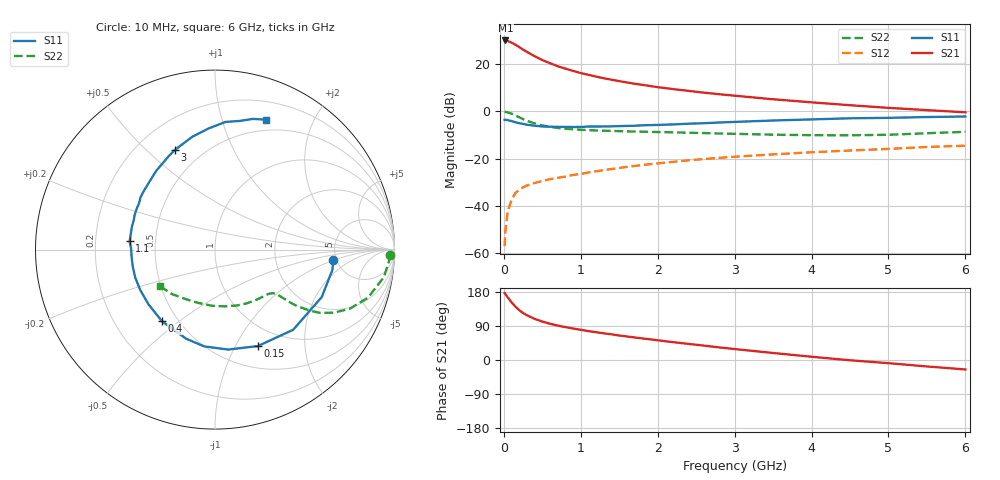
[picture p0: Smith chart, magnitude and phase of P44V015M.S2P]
! SIEMENS Small Signal Semiconductors
! BFP182
! Si NPN RF Bipolar Junction Transistor in SOT143
! VCE = 4 V  IC = 15 mA
! Common Emitter S-Parameters:  March  1996
# GHz  S  MA  R  50
!  f  S11  S21  S12  S22
! GHz  MAG  ANG  MAG  ANG  MAG  ANG  MAG  ANG
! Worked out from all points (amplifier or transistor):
!   36 points, 10 MHz to 6 GHz, reference 50 ohm
!   highest |S21| = 30.0 dB at 20 MHz (marker M1)
!   |S21| within 3 dB of that: start of sweep to 209.4 MHz
!   unconditionally stable (mu >= 1): 948.2 MHz to 5.389 GHz
!   at 250 MHz: K = 0.41, MSG = 29.2 dB, |S12| = -32.2 dB
!   at 1.4 GHz: K = 1.12, MAG = 16.8 dB, |S12| = -24.4 dB
!   at 6 GHz: K = 0.94, MSG = 7.1 dB, |S12| = -14.5 dB
!   S11 on the Smith chart (normalised r, x): 10 MHz: 4.71, -0.95; 150 MHz: 0.75, -1.24; 400 MHz: 0.41, -0.43; 1.1 GHz: 0.35, +0.04; 3 GHz: 0.36, +0.61; 6 GHz: 0.38, +1.40
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0.01  0.6616 -4.9  31.53 176.7  0.0014 86.1  0.9738 -1.7
0.02  0.6637 -9.9  31.71 174.3  0.0029 82.3  0.9722 -3.7
0.05  0.6508 -24.0  30.96 165.3  0.0077 81.1  0.9539 -9.2
0.1  0.6239 -45.7  28.52 152.2  0.0133 69.2  0.8938 -17.4
0.15  0.5882 -66.0  25.76 140.8  0.0187 63.0  0.8202 -23.7
0.2  0.5617 -82.5  22.98 131.5  0.022 57.8  0.7487 -28.0
0.25  0.5426 -96.4  20.29 124.0  0.0246 54.2  0.6851 -31.0
0.3  0.5218 -108.0  18.19 118.1  0.0269 51.9  0.6308 -32.7
0.4  0.4966 -126.5  14.71 108.5  0.0305 49.5  0.5541 -34.6
0.5  0.48 -140.6  12.18 101.3  0.0335 47.7  0.504 -35.2
0.6  0.4735 -151.5  10.47 95.7  0.0367 48.5  0.4698 -35.4
0.7  0.4711 -160.4  9.024 90.9  0.0392 48.8  0.446 -35.6
0.9  0.4665 -174.3  7.188 83.2  0.0451 49.4  0.417 -36.1
1.1  0.4781 174.3  5.936 76.2  0.0508 49.9  0.4 -37.5
1.5  0.4876 156.7  4.367 64.6  0.0635 50.3  0.3814 -41.5
1.8  0.5061 145.2  3.639 56.9  0.0729 49.4  0.3716 -45.7
2.2  0.5291 132.7  2.964 47.1  0.0854 47.0  0.3603 -52.2
3  0.5981 112.1  2.147 28.9  0.1096 41.1  0.3347 -68.4
3.5  0.6407 101.5  1.804 18.5  0.1228 36.9  0.3208 -80.4
4.5  0.7137 85.3  1.35 -0.7  0.1483 28.6  0.3113 -107.2
5.5  0.7583 73.8  1.063 -17.0  0.1765 21.0  0.3447 -134.0
6  0.7782 68.5  0.955 -25.0  0.1875 16.1  0.3688 -146.7
